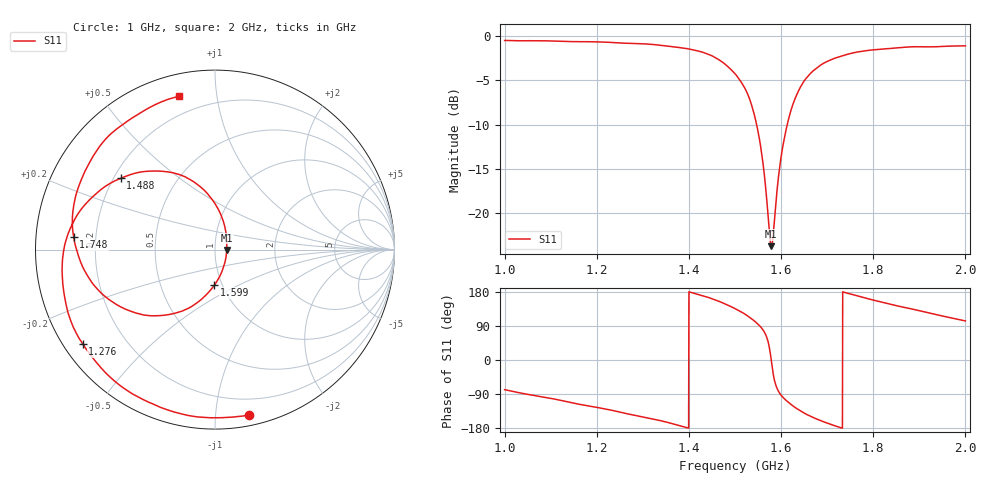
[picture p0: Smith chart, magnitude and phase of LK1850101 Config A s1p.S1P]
!Agilent Technologies,E5071C,
!Date: Sat May 06 11:13:36 2023
!Data & Calibration Information:
!Freq	S11:SOLT1(ON)
!PortZ  Port1:50+j0
!Above PortZ is port z conversion or system Z0 setting when saving the data.
!When reading, reference impedance value at option line is always used.
# Hz S dB R 50
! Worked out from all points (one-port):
!   1601 points, 1 GHz to 2 GHz, reference 50 ohm
!   lowest |S11| = -23.7 dB at 1.579 GHz (marker M1), VSWR 1.14, Z = 57 - j0.219 ohm
!   |S11| at or under -10 dB: 1.547 GHz to 1.613 GHz (66.48 MHz wide, 4.21 % of centre)
!   S11 on the Smith chart (normalised r, x): 1 GHz: 0.08, -1.23; 1.276 GHz: 0.05, -0.32; 1.488 GHz: 0.23, +0.32; 1.599 GHz: 0.92, -0.38; 1.748 GHz: 0.12, +0.04; 2 GHz: 0.11, +0.79
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1e9  -0.53 -78.3
1.069375e9  -0.56 -94.7
1.125e9  -0.62 -107.3
1.203125e9  -0.69 -125.7
1.25e9  -0.81 -137.4
1.27625e9  -0.86 -144.6
1.375e9  -1.30 -171.6
1.438125e9  -2.00 166.7
1.4875e9  -3.62 143.0
1.5e9  -4.27 135.7
1.525625e9  -6.35 117.9
1.54625e9  -9.85 98.6
1.56e9  -14.05 80.7
1.574375e9  -21.98 34.2
1.57875e9  -23.70 -1.7
1.583125e9  -22.29 -38.4
1.59875e9  -14.10 -90.9
1.610625e9  -10.64 -106.2
1.625e9  -7.84 -120.5
1.648125e9  -5.24 -138.6
1.683125e9  -3.41 -158.6
1.713125e9  -2.60 -172.1
1.7475e9  -2.04 175.0
1.75e9  -2.01 174.2
1.8e9  -1.59 158.2
1.875e9  -1.27 136.9
1.949375e9  -1.21 116.3
2e9  -1.13 103.2
